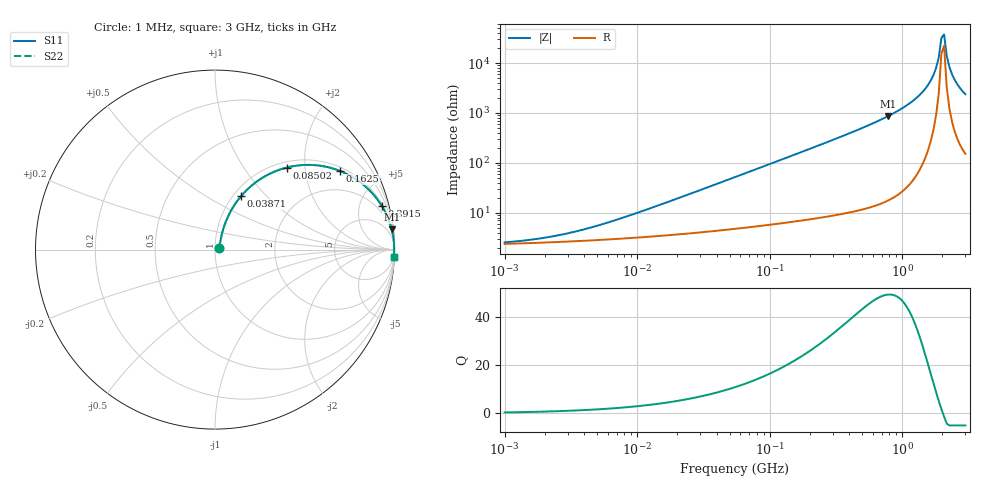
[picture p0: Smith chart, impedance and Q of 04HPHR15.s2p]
# MHz S MA R 50
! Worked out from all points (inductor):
!   174 points, 1 MHz to 3 GHz, reference 50 ohm
!   read as one part in series: L = 150 nH near 10.59 MHz
!   highest Q = 49.3 at 783.9 MHz (marker M1), where L = 176 nH
!   self-resonance near 1.978 GHz
!   S11 on the Smith chart (normalised r, x): 1 MHz: 1.05, +0.02; 38.71 MHz: 1.09, +0.73; 85.02 MHz: 1.11, +1.61; 162.5 MHz: 1.14, +3.08; 391.5 MHz: 1.20, +7.67; 3 GHz: 4, -48
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1  0.02493 21.1  0.9768 -0.5  0.9768 -0.5  0.02493 21.1
2.00209  0.03075 35.7  0.9752 -1.1  0.9752 -1.1  0.03075 35.7
3.8271  0.04399 50.9  0.9728 -2.0  0.9728 -2.0  0.04399 50.9
14.6467  0.1363 68.5  0.9584 -7.6  0.9584 -7.6  0.1363 68.5
38.7096  0.3325 64.0  0.9048 -19.3  0.9048 -19.3  0.3325 64.0
56.0545  0.4523 58.1  0.852 -26.8  0.852 -26.8  0.4523 58.1
85.016  0.6071 48.8  0.7546 -37.3  0.7546 -37.3  0.6071 48.8
162.512  0.8228 32.2  0.5332 -55.3  0.5332 -55.3  0.8228 32.2
214.526  0.8856 25.6  0.4328 -62.2  0.4328 -62.2  0.8856 25.6
391.532  0.9615 14.5  0.2508 -74.0  0.2508 -74.0  0.9615 14.5
783.883  0.9912 6.6  0.1141 -82.3  0.1141 -82.3  0.9912 6.6
821.013  0.9921 6.2  0.1072 -82.7  0.1072 -82.7  0.9921 6.2
1245.21  0.9972 3.0  0.05299 -85.4  0.05299 -85.4  0.9972 3.0
1569.41  0.9983 1.6  0.02717 -85.6  0.02717 -85.6  0.9983 1.6
1803.15  0.9985 0.7  0.01246 -82.8  0.01246 -82.8  0.9985 0.7
1888.56  0.9985 0.4  0.007672 -78.6  0.007672 -78.6  0.9985 0.4
1978.02  0.9985 0.2  0.003093 -60.6  0.003093 -60.6  0.9985 0.2
2071.71  0.9984 -0.1  0.002653 53.3  0.002653 53.3  0.9984 -0.1
2169.84  0.9983 -0.4  0.007157 76.2  0.007157 76.2  0.9983 -0.4
2272.62  0.9982 -0.7  0.01194 80.9  0.01194 80.9  0.9982 -0.7
2493.02  0.9978 -1.2  0.02166 83.5  0.02166 83.5  0.9978 -1.2
3000  0.9965 -2.4  0.04178 84.0  0.04178 84.0  0.9965 -2.4
